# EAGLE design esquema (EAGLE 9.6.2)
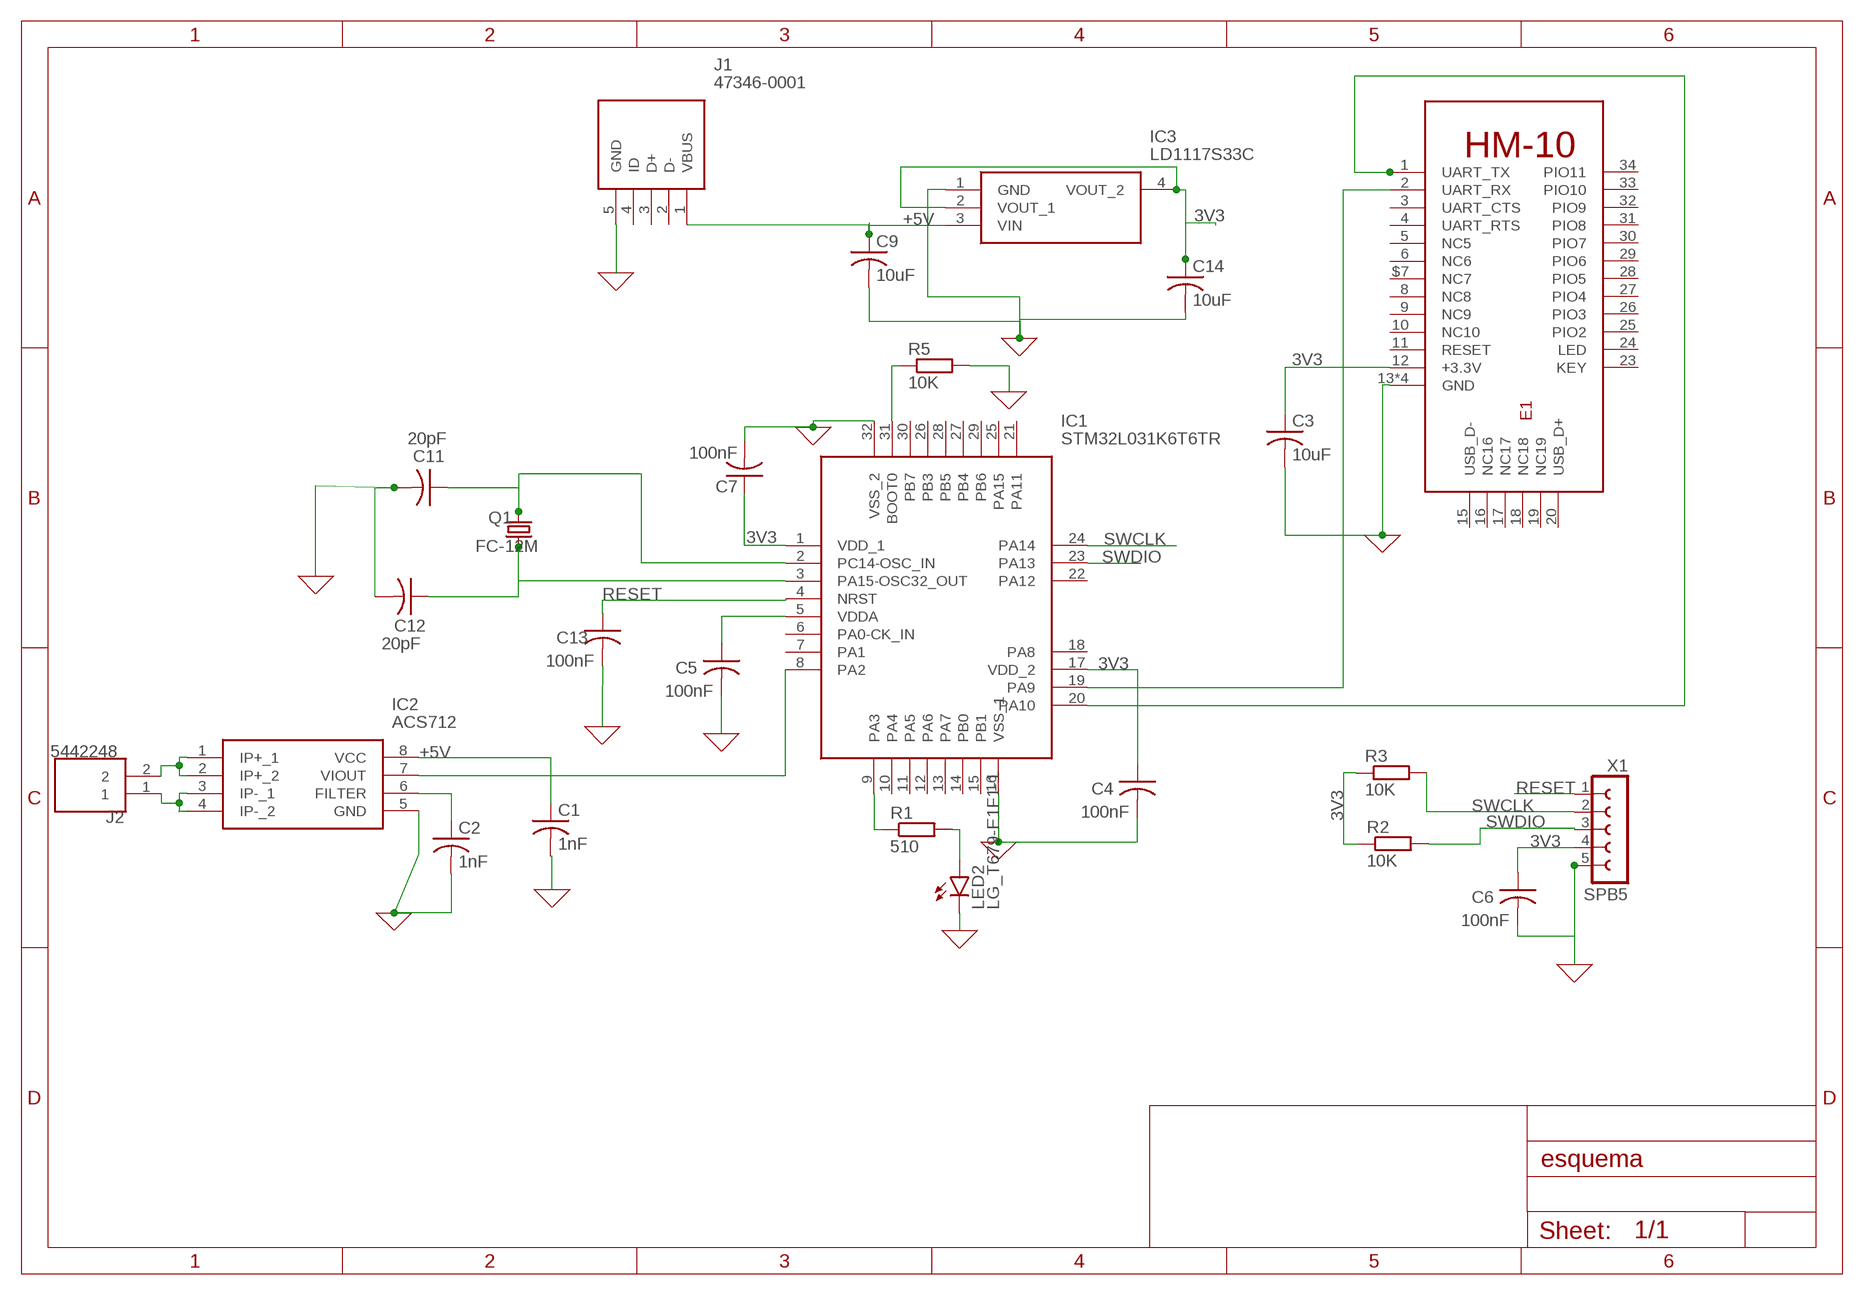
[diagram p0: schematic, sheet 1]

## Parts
C1  1nF  C-USC0805  [C0805]
C2  1nF  C-USC0805  [C0805]
C3  10uF  C-USC0805  [C0805]
C4  100nF  C-USC0805  [C0805]
C5  100nF  C-USC0805  [C0805]
C6  100nF  C-USC0805  [C0805]
C7  100nF  C-USC0805  [C0805]
C9  10uF  C-USC0805  [C0805]
C11  20pF  C-USC0805  [C0805]
C12  20pF  C-USC0805  [C0805]
C13  100nF  C-USC0805  [C0805]
C14  10uF  C-USC0805  [C0805]
E1  HM-10-BOARD  [26.9X13X2.2_BOARD]
IC1  STM32L031K6T6TR  [QFP80P900X900X160-32N]
IC2  ACS712  [SOIC127P600X175-8N]
IC3  LD1117S33C  [LD1117S33C]
J1  47346-0001  [47346-0001]
J2  5442248  [5442248]
LED2  LG_T679-E1F1-1  [PLCC2]
Q1  FC-12M  [FC-12M]
R1  510  R-EU_R0805  [R0805]
R2  10K  R-EU_R0805  [R0805]
R3  10K  R-EU_R0805  [R0805]
R5  10K  R-EU_R0805  [R0805]
X1  SPB5  [SPB5]

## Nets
3V3: C14.1 IC3.2(VOUT_1) IC3.4(VOUT_2)
+5V: C9.1 IC3.3(VIN) J1.1(VBUS)
GND: C1.2 C2.2 C3.2 C4.2 C5.2 C6.2 C7.2 C9.2 C11.2 C12.2 C13.2 C14.2 E1.13(GND) E1.14(GND) E1.21(GND) E1.22(GND) IC1.16(VSS_1) IC1.32(VSS_2) IC2.5(GND) IC3.1(GND) J1.5(GND) LED2.C R5.2 X1.5
N$1: IC1.8(PA2) IC2.7(VIOUT)
N$2: C11.1 IC1.2(PC14-OSC_IN) Q1.2
N$3: IC1.31(BOOT0) R5.1
N$4: C1.1 IC2.8(VCC)
N$5: C12.1 IC1.3(PA15-OSC32_OUT) Q1.1
N$6: IC1.23(PA13)
N$7: E1.2(UART_RX) IC1.19(PA9)
N$8: C13.1 IC1.4(NRST)
N$9: C2.1 IC2.6(FILTER)
N$10: C3.1 E1.12(+3.3V)
N$11: IC1.9(PA3) R1.1
N$12: C7.1 IC1.1(VDD_1)
N$13: C6.1 X1.4
N$14: C4.1 IC1.17(VDD_2)
N$15: LED2.A R1.2
N$16: C5.1 IC1.5(VDDA)
N$17: E1.1(UART_TX) IC1.20(PA10)
N$18: IC1.24(PA14)
N$19: IC2.1(IP+_1) IC2.2(IP+_2) J2.2
N$20: R2.1 R3.1
N$21: IC2.3(IP-_1) IC2.4(IP-_2) J2.1
RESET: X1.1
SWCLK: R3.2 X1.2
SWDIO: R2.2 X1.3
Unconnected: E1.3(UART_CTS) E1.4(UART_RTS) E1.5(NC5) E1.6(NC6) E1.8(NC8) E1.9(NC9) E1.10(NC10) E1.11(RESET) E1.15(USB_D-) E1.16(NC16) E1.17(NC17) E1.18(NC18) E1.19(NC19) E1.20(USB_D+) E1.23(KEY) E1.24(LED) E1.25(PIO2) E1.26(PIO3) E1.27(PIO4) E1.28(PIO5) E1.29(PIO6) E1.30(PIO7) E1.31(PIO8) E1.32(PIO9) E1.33(PIO10) E1.34(PIO11) E1.$7(NC7) IC1.6(PA0-CK_IN) IC1.7(PA1) IC1.10(PA4) IC1.11(PA5) IC1.12(PA6) IC1.13(PA7) IC1.14(PB0) IC1.15(PB1) IC1.18(PA8) IC1.21(PA11) IC1.22(PA12) IC1.25(PA15) IC1.26(PB3) IC1.27(PB4) IC1.28(PB5) IC1.29(PB6) IC1.30(PB7) J1.2(D-) J1.3(D+) J1.4(ID)

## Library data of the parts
C1-C7 C9 C11-C14 = rcl:C-US: CAPACITOR, American symbol; SPICEPREFIX: C
E1 = hm10:HM-10: HM Bluetooth module use TI CC2540 or CC2541, Master and slave roles in one, transmission version and remote control version and PIO state acquisition functions in one, Support the AT command modify module parameters, Convenient and flexible.
IC1 = STM32L031K6T6TR:STM32L031K6T6TR: STMICROELECTRONICS - STM32L031K6T6TR - ARM MCU, STM32 Family STM32L0 Series Microcontrollers, ARM Cortex-M0+, 32bit, 32 MHz, 32 KB, 8 KB Source: Datasheet; ARROW_PART_NUMBER: STM32L031K6T6TR; ARROW_PRICE-STOCK: https://www.arrow.com/en/products/stm32l031k6t6tr/stmicroelectronics; DESCRIPTION: STMICROELECTRONICS - STM32L031K6T6TR - ARM MCU, STM32 Family STM32L0 Series Microcontrollers, ARM Cortex-M0+, 32bit, 32 MHz, 32 KB, 8 KB; HEIGHT: 1.6mm; MANUFACTURER_NAME: STMicroelectronics; MANUFACTURER_PART_NUMBER: STM32L031K6T6TR; MOUSER_PART_NUMBER: 511-STM32L031K6T6TR; MOUSER_PRICE-STOCK: https://www.mouser.co.uk/ProductDetail/STMicroelectronics/STM32L031K6T6TR/?qs=xwQlLnDx56Cmxri8cgW0QQ%3D%3D
IC2 = ACS712:ACS712: Fully Integrated, Hall Effect-Based Linear Current Sensor IC with 2.1 kVRMS Isolation and a Low-Resistance Current Conductor Source: Datasheet; DESCRIPTION: Fully Integrated, Hall Effect-Based Linear Current Sensor IC with 2.1 kVRMS Isolation and a Low-Resistance Current Conductor; HEIGHT: 1.75mm; MANUFACTURER_NAME: Allegro Microsystems; MANUFACTURER_PART_NUMBER: ACS712
IC3 = LD1117S33C:LD1117S33C: IC: voltage regulator; LDO, linear, fixed; 3.3V; 0.95A; SOT223; SMD Source: Datasheet; DESCRIPTION: IC: voltage regulator; LDO, linear, fixed; 3.3V; 0.95A; SOT223; SMD; HEIGHT: 1.8mm; MANUFACTURER_NAME: STMicroelectronics; MANUFACTURER_PART_NUMBER: LD1117S33C
J1 = 47346-0001:47346-0001: Micro USB B Receptacle Bottom Mount Assy Molex Right Angle SMT Type B Version 2.0 Micro USB Connector Socket, 30 V ac, 1A 47352 MICRO-USB Source: Datasheet; DESCRIPTION: Micro USB B Receptacle Bottom Mount Assy Molex Right Angle SMT Type B Version 2.0 Micro USB Connector Socket, 30 V ac, 1A 47352 MICRO-USB; HEIGHT: mm; MANUFACTURER_NAME: Molex; MANUFACTURER_PART_NUMBER: 47346-0001; MOUSER_PART_NUMBER: 538-47346-0001; MOUSER_PRICE-STOCK: https://www.mouser.co.uk/ProductDetail/Molex/47346-0001?qs=c2CV6XM0DweJBWaSeyWeCw%3D%3D
J2 = 5442248:5442248: Fixed Terminal Blocks BC-350X9- 2 GN 3.5 MM PITCH; ARROW_PART_NUMBER: 5442248; ARROW_PRICE-STOCK: https://www.arrow.com/en/products/5442248/phoenix-contact; DESCRIPTION: Fixed Terminal Blocks BC-350X9- 2 GN 3.5 MM PITCH; HEIGHT: 8.65mm; MANUFACTURER_NAME: Phoenix Contact; MANUFACTURER_PART_NUMBER: 5442248; MOUSER_PART_NUMBER: 651-5442248; MOUSER_PRICE-STOCK: https://www.mouser.co.uk/ProductDetail/Phoenix-Contact/5442248?qs=9Y9qB%2FCsC3kNHrXWmi1dGA%3D%3D
LED2 = led:*_T679-?-1: LC TOPLED® Low Current LED; COLOR: green
Q1 = crystal:FC-12M: kHz RANGE CRYSTAL UNIT
R1-R3 R5 = rcl:R-EU_: RESISTOR, European symbol; SPICEPREFIX: R
X1 = con-hirschmann:SPB5: CONNECTOR 5 pins; OC_FARNELL: unknown; OC_NEWARK: unknown

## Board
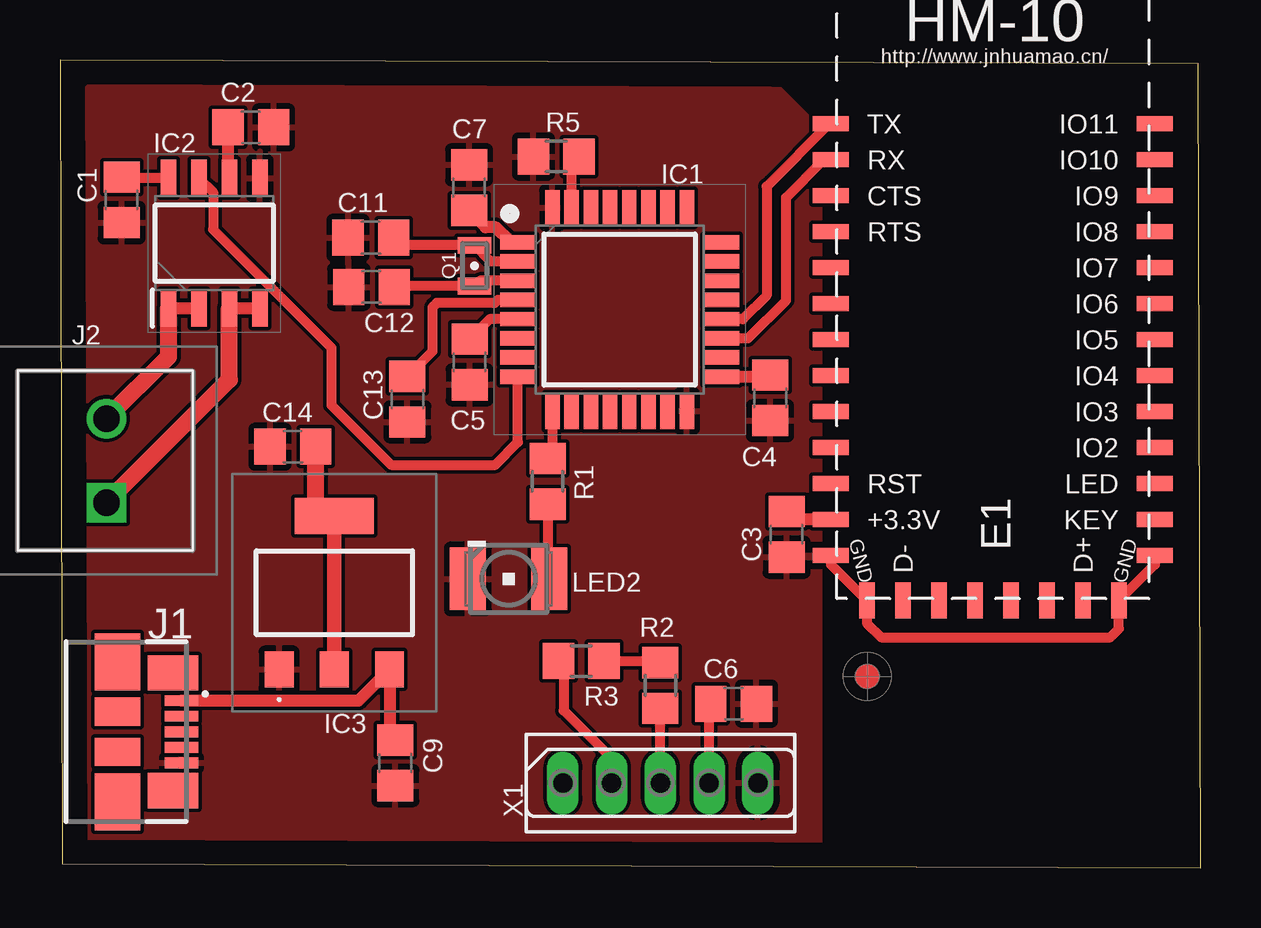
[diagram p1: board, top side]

Size 47.52 x 33.67 mm. Coordinates in mm from the lower left corner, seen from the top.
Outline: 0.1,0.15 47.52,0 47.42,33.52 0,33.67 0.1,0.15
Copper layers (1*16): Top 0.035mm / dielectric 1.5mm / Bottom 0.035mm
Design rules "default": minimum track width 6mil, minimum drill 0.35mm, track to track 6mil, track to pad 6mil, pad to pad 6mil, via to via 6mil, smd to smd 6mil, copper to edge 40mil, drill to drill 6mil, minimum pad ring 10mil, minimum via ring 8mil, stop-mask expansion 4mil, vias tented up to drill 0mil, thermal gap 10mil

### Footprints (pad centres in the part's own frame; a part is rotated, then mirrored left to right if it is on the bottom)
C0805 = smd 1.3 x 1.5: 1 -0.95,0; 2 0.95,0
26.9X13X2.2_BOARD = smd 1.5 x 0.635: 1 -7.5,0; 2 -7.5,-1.5; 3 -7.5,-3; 4 -7.5,-4.5; 5 -7.5,-6; 6 -7.5,-7.5; 8 -7.5,-10.5; 9 -7.5,-12; 10 -7.5,-13.5; 11 -7.5,-15; 12 -7.5,-16.5; 13 -7.5,-18; 22 6,-18; 23 6,-16.5; 24 6,-15; 25 6,-13.5; 26 6,-12; 27 6,-10.5; 28 6,-9; 29 6,-7.5; 30 6,-6; 31 6,-4.5; 32 6,-3; 33 6,-1.5; 34 6,0; $7 -7.5,-9 | smd 0.635 x 1.5: 14 -6,-19.875; 15 -4.5,-19.875; 16 -3,-19.875; 17 -1.5,-19.875; 18 0,-19.875; 19 1.5,-19.875; 20 3,-19.875; 21 4.5,-19.875
QFP80P900X900X160-32N = smd 1.475 x 0.6: 1 -4.238,2.8; 2 -4.238,2; 3 -4.238,1.2; 4 -4.238,0.4; 5 -4.238,-0.4; 6 -4.238,-1.2; 7 -4.238,-2; 8 -4.238,-2.8; 17 4.238,-2.8; 18 4.238,-2; 19 4.238,-1.2; 20 4.238,-0.4; 21 4.238,0.4; 22 4.238,1.2; 23 4.238,2; 24 4.238,2.8 | smd 0.6 x 1.475: 9 -2.8,-4.238; 10 -2,-4.238; 11 -1.2,-4.238; 12 -0.4,-4.238; 13 0.4,-4.238; 14 1.2,-4.238; 15 2,-4.238; 16 2.8,-4.238; 25 2.8,4.238; 26 2,4.238; 27 1.2,4.238; 28 0.4,4.238; 29 -0.4,4.238; 30 -1.2,4.238; 31 -2,4.238; 32 -2.8,4.238
SOIC127P600X175-8N = smd 1.525 x 0.65: 1 -2.712,1.905; 2 -2.712,0.635; 3 -2.712,-0.635; 4 -2.712,-1.905; 5 2.712,-1.905; 6 2.712,-0.635; 7 2.712,0.635; 8 2.712,1.905
LD1117S33C = smd 1.2 x 1.5: 1 -2.3,-3.2; 2 0,-3.2; 3 2.3,-3.2 | smd 3.3 x 1.5: 4 0,3.2
47346-0001 = smd 0.45 x 1.38: 1 1.3,-4.81; 2 0.65,-4.81; 3 0,-4.81; 4 -0.65,-4.81; 5 -1.3,-4.81 | smd 1.475 x 2.1: 6 -2.453,-4.45; 7 2.453,-4.45 | smd 1.175 x 1.9: 8 0.838,-2.15; 9 -0.838,-2.15 | smd 2.375 x 1.9: 10 2.913,-2.15; 11 -2.913,-2.15
5442248 = drill 1.1 pad 1.65 square: 1 0,0 | drill 1.1 pad 1.65: 2 3.5,0
PLCC2 = smd 2.6 x 1.5: A 0,1.7; C 0,-1.7
FC-12M = smd 0.7 x 1.4: 1 -0.85,0; 2 0.85,0
R0805 = smd 1.3 x 1.5: 1 -0.95,0; 2 0.95,0
SPB5 = drill 0.813 long: 1 -4.064,0; 2 -2.032,0; 3 0,0; 4 2.032,0; 5 4.064,0

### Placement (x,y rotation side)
C1  2.57,27.84 270 top
C2  7.95,30.86 0 top
C3  30.28,13.89 270 top
C4  29.59,19.58 270 top
C5  17.07,21.08 270 top
C6  28.07,6.83 0 top
C7  17.04,28.35 90 top
C9  13.97,4.37 270 top
C11  12.95,26.26 180 top
C12  12.98,24.21 180 top
C13  14.48,19.53 270 top
C14  9.7,17.55 180 top
E1  39.62,31.01 0 top
IC1  23.32,23.27 0 top
IC2  6.43,26.04 90 top
IC3  11.43,11.46 0 top
J1  0.25,5.66 90 top
J2  1.93,15.21 90 top
LED2  18.69,12.04 270 top
Q1  17.27,25.1 90 top
R1  20.32,16.1 270 top
R2  25.02,7.59 270 top
R3  21.72,8.61 180 top
R5  20.68,29.64 180 top
U$1  [FIDUCIAL_G10]  33.63,7.98 0 top
X1  25.02,3.53 0 top

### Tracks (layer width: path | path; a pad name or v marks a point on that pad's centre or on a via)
3V3
  Top 0.508: IC3.4 10.65,15.43
  Top 0.61: IC3.2 IC3.4
  Top 0.711: 10.65,15.43 C14.1
+5V
  Top 0.508: J1.1 12.44,6.96 IC3.3 13.73,5.56 C9.1
GND
  Top 0.406: E1.22 45.62,12.64 E1.21 44.12,9.96 43.76,9.6 34.21,9.6 33.62,10.19 E1.14 32.12,12.64 E1.13
  pour Top: 1.32,32.74 1.5,32.92 29.59,32.92 31.7,30.81 31.7,0.69 0.84,0.69 0.71,0.56 0.71,32.11 0.71,32.16 0.74,32.16
N$1
  Top 0.406: IC2.7 6.38,28.16 6.38,26.6 11.3,21.68 11.3,19.28 13.79,16.79 18.14,16.79 19.08,17.73 IC1.8
N$2
  Top 0.406: C11.1 14.22,25.94 Q1.2 17.95,25.27 IC1.2
N$3
  Top 0.406: IC1.31 21.32,29.33 R5.1
N$4
  Top 0.406: IC2.8 2.61,28.75 C1.1
N$5
  Top 0.406: C12.1 13.97,24.24 Q1.1 17.49,24.47 IC1.3
N$7
  Top 0.406: IC1.19 28.67,22.07 30.25,23.65 30.25,27.94 31.82,29.51 E1.2
N$8
  Top 0.406: IC1.4 18.25,23.67 18.12,23.54 15.69,23.54 15.52,23.37 15.52,21.52 C13.1
N$9
  Top 0.508: IC2.6 7,28.81 C2.1
N$10
  Top 0.508: E1.12 30.61,14.51 C3.1
N$11
  Top 0.406: IC1.9 20.52,17.25 R1.1
N$12
  Top 0.508: C7.1 17.74,26.7 18.14,26.7 18.78,26.07 IC1.1
N$13
  Top 0.406: X1.4 27.05,6.77 C6.1
N$14
  Top 0.508: IC1.17 29.52,20.47 C4.1
N$15
  Top 0.406: R1.2 20.32,12.11 LED2.A
N$16
  Top 0.406: IC1.5 17.9,22.87 C5.1
N$17
  Top 0.406: E1.1 32.05,31.01 29.44,28.4 29.44,23.85 28.45,22.86 IC1.20
N$19
  Top 0.508: IC2.1 IC2.2
  Top 0.711: J2.2 4.52,21.31 IC2.1
N$20
  Top 0.406: R3.1 24.95,8.61 R2.1
N$21
  Top 0.508: IC2.3 IC2.4
  Top 0.711: J2.1 7.06,20.35 IC2.3
SWCLK
  Top 0.406: R3.2 20.98,8.4 20.98,6.55 22.99,4.55 X1.2
SWDIO
  Top 0.406: X1.3 R2.2

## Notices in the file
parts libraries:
dicons: Copyright (C) 2004, Bob Starr (rtzaudio@mindspring.com)
